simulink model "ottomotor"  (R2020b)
settings: Solver=ode45  StartTime=0.0  StopTime=0.02  FixedStep=0.01  RelTol=1e-6  AbsTol=1e-10
model workspace (MAT data in the model file):
  Pe = 0.65
  Qges = 91
  R = 287
  TW = 300
  Vc = 5.15e-06
  a = 6.91
  alphaW = 350
  be = 400
  cp = 1050
  d = 0.039
  dphiB = 1.04716666667
  e = 8
  h = 0.029
  l = 0.052
  lam = 0.25
  m = 2
  mL = 3.95e-05
  n = 3350
  r = 0.013

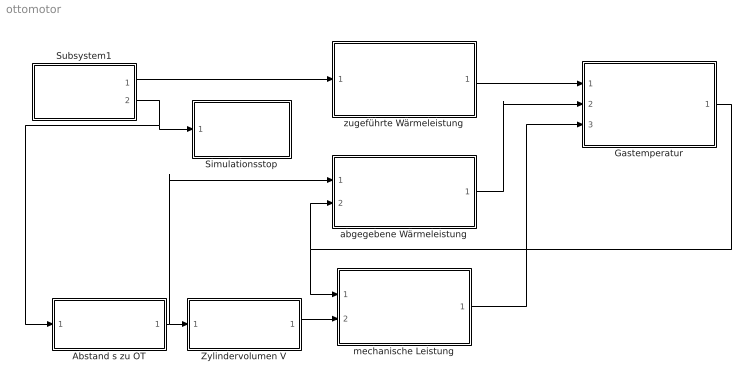
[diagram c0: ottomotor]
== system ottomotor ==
  Abstand s zu OT : Subsystem
  Gastemperatur : Subsystem
  Simulationsstop : Subsystem
  Subsystem1 : Subsystem
  Zylindervolumen V : Subsystem
  abgegebene Wärmeleistung : Subsystem
  mechanische Leistung : Subsystem
  zugeführte Wärmeleistung : Subsystem
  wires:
  Gastemperatur/1(T) -> mechanische Leistung/1(T), abgegebene Wärmeleistung/2(T)
  Zylindervolumen V/1(V) -> mechanische Leistung/2(V)
  abgegebene Wärmeleistung/1(Q_dot_ab) -> Gastemperatur/2(Q_dot_ab)
  Abstand s zu OT/1(s) -> abgegebene Wärmeleistung/1(s), Zylindervolumen V/1(In1)
  mechanische Leistung/1(W_dot) -> Gastemperatur/3(W_dot)
  zugeführte Wärmeleistung/1(Q_dot_zu) -> Gastemperatur/1(Q_dot_zu)
  Subsystem1/1(Out2) -> zugeführte Wärmeleistung/1(phi)
  Subsystem1/2(phi) -> Abstand s zu OT/1(phi), Simulationsstop/1(phi)

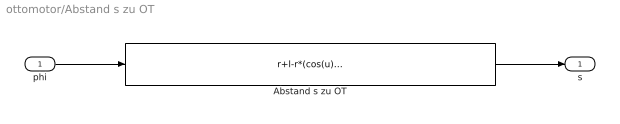
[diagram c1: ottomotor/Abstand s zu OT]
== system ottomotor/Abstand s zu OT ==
  phi : Inport
  Abstand s zu OT : Fcn  Expr=r+l-r*(cos(u)+1/lam-lam/4+lam/4*cos(2*u))
  s : Outport
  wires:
  phi/1 -> Abstand s zu OT/1
  Abstand s zu OT/1 -> s/1

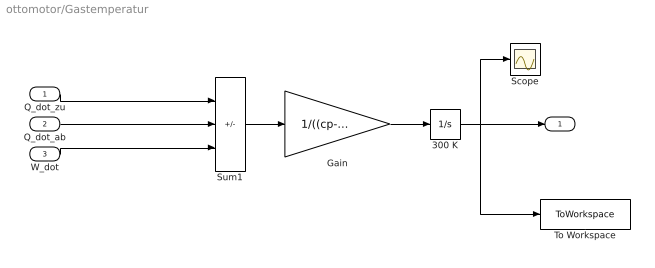
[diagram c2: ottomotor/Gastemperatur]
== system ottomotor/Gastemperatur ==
  Q_dot_zu : Inport
  Q_dot_ab : Inport  Port=2
  W_dot : Inport  Port=3
  300 K : Integrator  InitialCondition=300
  Gain : Gain  Gain=1/((cp-R)*mL)  SaturateOnIntegerOverflow=on
  Scope : Scope
  Sum1 : Sum  Inputs=+--  SaturateOnIntegerOverflow=on
  To Workspace : ToWorkspace  VariableName=T  SaveFormat=Timeseries  SampleTime=-1
  T : Outport
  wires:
  Sum1/1 -> Gain/1
  W_dot/1 -> Sum1/3
  Gain/1 -> 300 K/1
  Q_dot_zu/1 -> Sum1/1
  Q_dot_ab/1 -> Sum1/2
  300 K/1 -> To Workspace/1, Scope/1, T/1

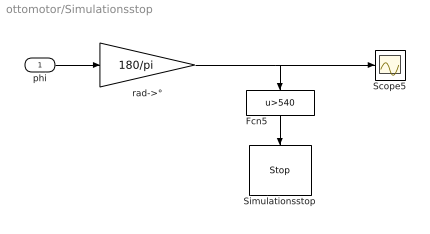
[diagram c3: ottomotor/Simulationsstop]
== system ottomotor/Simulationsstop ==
  phi : Inport
  Fcn5 : Fcn  Expr=u>540
  Scope5 : Scope
  Simulationsstop : Stop
  rad->° : Gain  Gain=180/pi  SaturateOnIntegerOverflow=on
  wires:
  phi/1 -> rad->°/1
  Fcn5/1 -> Simulationsstop/1
  rad->°/1 -> Fcn5/1, Scope5/1

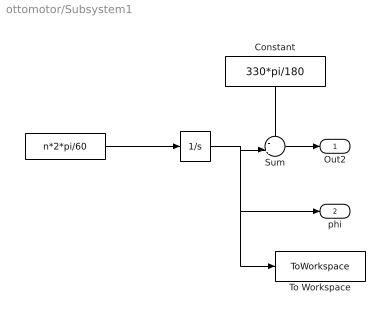
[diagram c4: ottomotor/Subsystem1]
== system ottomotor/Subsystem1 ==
  " " : Integrator  InitialCondition=pi
  "  " : Constant  Value=n*2*pi/60
  Constant : Constant  Value=330*pi/180
  Sum : Sum  Inputs=-+|  SaturateOnIntegerOverflow=on
  To Workspace : ToWorkspace  VariableName=Phi  SaveFormat=Timeseries  SampleTime=-1
  Out2 : Outport
  phi : Outport  Port=2
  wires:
  " "/1 -> Sum/2, To Workspace/1, phi/1
  Constant/1 -> Sum/1
  "  "/1 -> " "/1
  Sum/1 -> Out2/1

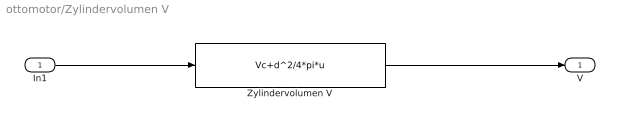
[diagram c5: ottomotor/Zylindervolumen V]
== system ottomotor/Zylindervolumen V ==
  In1 : Inport
  Zylindervolumen V : Fcn  Expr=Vc+d^2/4*pi*u
  V : Outport
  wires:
  In1/1 -> Zylindervolumen V/1
  Zylindervolumen V/1 -> V/1

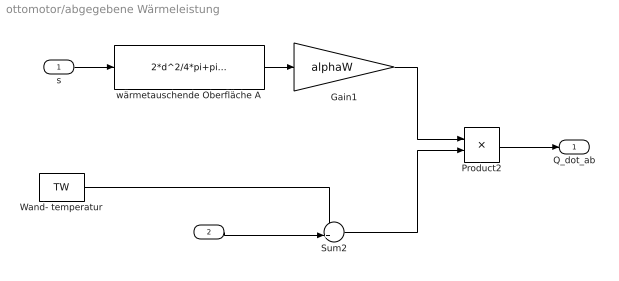
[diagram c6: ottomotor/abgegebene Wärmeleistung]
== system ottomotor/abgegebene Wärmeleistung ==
  s : Inport
  T : Inport  Port=2
  Gain1 : Gain  Gain=alphaW  SaturateOnIntegerOverflow=on
  Product2 : Product  SaturateOnIntegerOverflow=on
  Sum2 : Sum  Inputs=-+|  SaturateOnIntegerOverflow=on
  Wand- temperatur : Constant  Value=TW
  wärmetauschende Oberfläche A : Fcn  Expr=2*d^2/4*pi+pi*d*u
  Q_dot_ab : Outport
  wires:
  wärmetauschende Oberfläche A/1 -> Gain1/1
  Gain1/1 -> Product2/1
  s/1 -> wärmetauschende Oberfläche A/1
  Wand- temperatur/1 -> Sum2/1
  Sum2/1 -> Product2/2
  T/1 -> Sum2/2
  Product2/1 -> Q_dot_ab/1

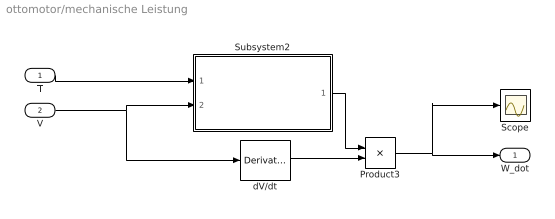
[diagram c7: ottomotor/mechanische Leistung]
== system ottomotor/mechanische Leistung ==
  T : Inport
  V : Inport  Port=2
  Product3 : Product  SaturateOnIntegerOverflow=on
  Scope : Scope
  Subsystem2 : Subsystem
  dV/dt : Derivative
  W_dot : Outport
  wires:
  T/1 -> Subsystem2/1(T)
  Subsystem2/1(pz) -> Product3/1
  dV/dt/1 -> Product3/2
  V/1 -> dV/dt/1, Subsystem2/2(V)
  Product3/1 -> Scope/1, W_dot/1

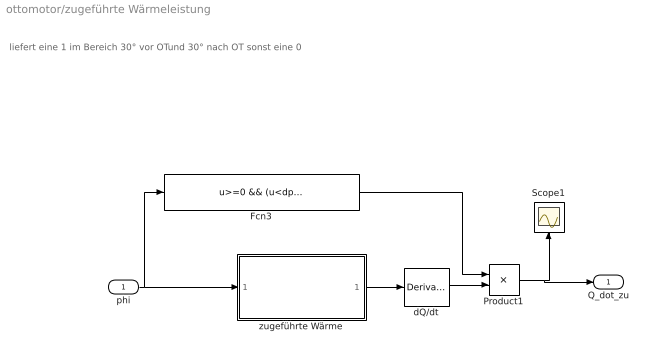
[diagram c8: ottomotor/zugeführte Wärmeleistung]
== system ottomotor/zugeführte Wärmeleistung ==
  note: liefert eine 1 im Bereich 30° vor OTund 30° nach OT sonst eine 0
  phi : Inport
  Fcn3 : Fcn  Expr=u>=0 && (u<dphiB)
  Product1 : Product  SaturateOnIntegerOverflow=on
  Scope1 : Scope
  dQ/dt : Derivative
  zugeführte Wärme : Subsystem
  Q_dot_zu : Outport
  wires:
  zugeführte Wärme/1(Q) -> dQ/dt/1
  Product1/1 -> Q_dot_zu/1, Scope1/1
  dQ/dt/1 -> Product1/2
  phi/1 -> Fcn3/1, zugeführte Wärme/1(phi)
  Fcn3/1 -> Product1/1

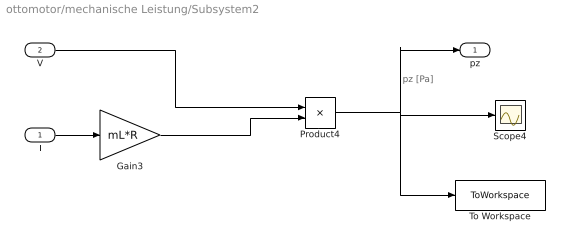
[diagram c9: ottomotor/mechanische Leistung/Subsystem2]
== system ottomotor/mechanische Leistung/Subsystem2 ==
  note: pz [Pa]
  T : Inport
  V : Inport  Port=2
  Gain3 : Gain  Gain=mL*R  SaturateOnIntegerOverflow=on
  Product4 : Product  Inputs=/*  SaturateOnIntegerOverflow=on
  Scope4 : Scope
  To Workspace : ToWorkspace  VariableName=p  SaveFormat=Timeseries  SampleTime=-1
  pz : Outport
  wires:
  V/1 -> Product4/1
  Product4/1 -> To Workspace/1, pz/1, Scope4/1
  Gain3/1 -> Product4/2
  T/1 -> Gain3/1

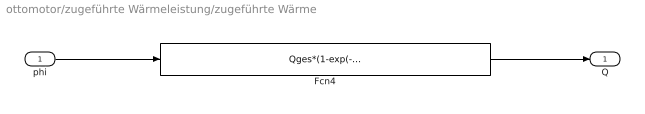
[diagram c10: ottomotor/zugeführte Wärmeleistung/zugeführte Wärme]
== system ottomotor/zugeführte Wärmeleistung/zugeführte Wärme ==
  phi : Inport
  Fcn4 : Fcn  Expr=Qges*(1-exp(-a*(u/dphiB)^(m+1)))
  Q : Outport
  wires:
  phi/1 -> Fcn4/1
  Fcn4/1 -> Q/1
